| IBIS file stm32mp251_253_255_257_vfbga361.ibs
[IBIS ver] 5.1
[File name] stm32mp251_253_255_257_vfbga361.ibs
[File Rev] 1.3
[Date] 09-10-2025
[Source] Data Created at STMicroelectronics
[Notes]  File originated from ELDO simulations.
[Disclaimer]  This information is for modeling purpose only and is
   not guaranted. The information is subject to change without
   notice.
[Copyright] Copyright 2025 STMicroelectronics Inc.
|   Component stm32mp251_253_255_257_vfbga361
[Component] stm32mp251_253_255_257_vfbga361
[Manufacturer] STMicroelectronics
[Package]
| variable   typ   min   max
R_pkg   0.0   0.0   0.0
L_pkg   0.0H   0.0H   0.0H
C_pkg   0.0F   0.0F   0.0F
[Pin]  signal_name   model_name   R_pin   L_pin   C_pin
A1 VSS gnd
A10 PD2 io8_tt
A11 PD15 io8_tt_i3c
A12 PD6 io8_tt
A13 PD14 io8_tt_i3c
A14 PE2 io8_tt
A15 PE3 io8_tt
A16 PE13 io8_tt
A17 DDR_DQ11 mal4drv27_PAD
A18 DDR_DQ9 mal4drv27_PAD
A19 VSS gnd
A2 DSI_D3P DPHY_IBIS
A3 DSI_D2P DPHY_IBIS
A4 DSI_CKN DPHY_IBIS
A5 DSI_D0N DPHY_IBIS
A6 DSI_D1N DPHY_IBIS
A7 PB8 io8_tt
A8 PB9 io8_tt
A9 PB3 io8_tt
B1 VDDCSI nc
B10 PD11 io8_tt_i3c
B11 B11 nc
B12 PD5 io8_tt
B13 PE0 io8_tt
B14 PE4 io8_tt
B15 PE8 io8_tt
B16 PE11 io8_tt
B17 DDR_DQ10 mal4drv27_PAD
B18 DDR_DQS1N mal4drv27_PAD
B19 DDR_DQS1P mal4drv27_PAD
B2 DSI_D3N DPHY_IBIS
B3 DSI_D2N DPHY_IBIS
B4 DSI_CKP DPHY_IBIS
B5 DSI_D0P DPHY_IBIS
B6 DSI_D1P DPHY_IBIS
B7 PB11 io8_tt
B8 PB0 io8_tt
B9 PB5 io8_tt_i3c
C1 CSI_CKP DPHY_IBIS_L1
C10 PD9 io8_tt
C11 PD0 io8_tt
C12 PD4 io8_tt
C13 PE1 io8_tt
C14 PE5 io8_tt
C15 PE7 io8_tt
C16 PE12 io8_tt
C17 DDR_DQ8 mal4drv27_PAD
C18 DDR_DQ15 mal4drv27_PAD
C19 DDR_DQM1 mal4drv27_PAD
C2 CSI_CKN DPHY_IBIS_L1
C3 VSS gnd
C4 DSI_REXT nc
C5 VDDA18DSI power
C6 VDDDSI nc
C7 VSS gnd
C8 PB6 io8_tt
C9 PB4 io8_tt_i3c
D1 CSI_D1P DPHY_IBIS_L1
D10 VDDIO1 power
D11 PD10 io8_tt_i3c
D12 PD7 io8_tt
D13 VSS gnd
D14 PE15 io8_tt
D15 PE10 io8_tt
D16 VDDA18DDR nc
D17 DDR_DQ14 mal4drv27_PAD
D18 DDR_DQ13 mal4drv27_PAD
D19 DDR_DQ12 mal4drv27_PAD
D2 CSI_D1N DPHY_IBIS_L1
D3 VDDA18CSI power
D4 D4 nc
D5 D5 nc
D6 VDDIO4 power
D7 PB7 io8_tt
D8 PD3 io8_tt
D9 PB1 io8_tt
E1 CSI_D0N DPHY_IBIS_L1
E10 VDDIO3 power
E11 PD8 io8_tt
E12 PB10 io8_tt
E13 VDDCPU nc
E14 PB12 io8_tt
E15 VDDA18PLL1 nc
E16 VSS gnd
E17 DDR_RESETN nc
E18 DDR_A9 mal4drv20_PAD
E19 DDR_A20 mal4drv20_PAD
E2 CSI_D0P DPHY_IBIS_L1
E3 CSI_REXT nc
E4 PG15 io8_tt
E5 PG8 io8_tt
E6 VDDIO4 power
E7 PG7 io8_tt
E8 VSS gnd
E9 PB2 io8_tt
F1 LVDS1_D0N nc
F10 VDDIO3 power
F11 VSS gnd
F12 F12 nc
F13 VSS gnd
F14 PE6 io8_tt
F15 PE9 io8_tt
F16 VDDQDDR power
F17 DDR_A0 mal4drv20_PAD
F18 DDR_A11 mal4drv20_PAD
F19 DDR_A21 mal4drv20_PAD
F2 LVDS1_D0P nc
F3 LVDS1_D1N nc
F4 LVDS1_D1P nc
F5 PG10 io8_tt
F6 VSS gnd
F7 PG11 io8_tt
F8 VDDIO2 power
F9 PD1 io8_tt
G1 G1 nc
G10 VDDCORE nc
G11 VSS gnd
G12 PH4 io8_tt
G13 VDDCPU nc
G14 PE14 io8_tt
G15 PB13 io8_tt
G16 DDR_ZQ nc
G17 DDR_A1 mal4drv20_PAD
G18 DDR_A10 mal4drv20_PAD
G19 DDR_A22 mal4drv20_PAD
G2 PG9 io8_tt
G3 LVDS1_D2N nc
G4 LVDS1_D2P nc
G5 PF15 io8_tt
G6 VDDA18PLL2 nc
G7 PF14 io8_tt
G8 VSS gnd
G9 PD13 io8_tt
H1 PI0 io8_tt
H10 VSS gnd
H11 VDDCORE nc
H12 PG3 io8_tt
H13 VSS gnd
H14 PD12 io8_tt
H15 PB14 io8_tt
H16 VSS gnd
H17 DDR_A25 mal4drv20_PAD
H18 DDR_A8 mal4drv20_PAD
H19 DDR_A23 mal4drv20_PAD
H2 PF13 io8_tt
H3 LVDS1_D4N nc
H4 LVDS1_D4P nc
H5 PG14 io8_tt
H6 VDDA18PLL3 nc
H7 PG12 io8_tt
H8 VDD power
H9 PI3 io8_tt
J1 VDDLVDS nc
J10 VDDCORE nc
J11 VSS gnd
J12 PA5 io8_tt
J13 VDDCPU nc
J14 VSS gnd
J15 PB15 io8_tt
J16 VDDQDDR power
J17 DDR_A2 mal4drv20_PAD
J18 DDR_A13 mal4drv20_PAD
J19 DDR_A3 mal4drv20_PAD
J2 LVDS1_D3N nc
J3 LVDS1_D3P nc
J4 VDDA18LVDS power
J5 PI2 io8_tt
J6 VSS gnd
J7 PG13 io8_tt_i3c
J8 VSS gnd
J9 PI1 io8_tt_i3c
K1 PG5 io8_tt_i3c
K10 VSS gnd
K11 VDDCORE nc
K12 PA9 io8_tt
K13 VSS gnd
K14 PH3 io8_tt_i3c
K15 PA7 io8_tt
K16 VSS gnd
K17 DDR_VREF nc
K18 DDR_A14 mal4drv20_PAD
K19 DDR_A26 mal4drv20_PAD
K2 PG6 io8_tt_i3c
K3 PZ6 io8_tt
K4 VSS gnd
K5 VSS gnd
K6 K6 nc
K7 K7 nc
K8 VDD power
K9 PA8 io8_tt_i3c
L1 PZ7 io8_tt
L10 VDDCORE nc
L11 VSS gnd
L12 PH7 io8_tt_i3c
L13 VDDCPU nc
L14 PH2 io8_tt_i3c
L15 PH6 io8_tt_i3c
L16 VDDQDDR power
L17 DDR_A5 mal4drv20_PAD
L18 DDR_A15 mal4drv20_PAD
L19 DDR_A27 mal4drv20_PAD
L2 PZ9 io8_tt_i3c
L3 PZ8 io8_tt
L4 PZ4 io8_tt_i3c
L5 PZ0 io8_tt_i3c
L6 VDD power
L7 PF12 io8_tt
L8 VSS gnd
L9 PF10 io8_tt
M1 OSC32_OUT isudq_tt
M10 VSS gnd
M11 VDDGPU nc
M12 PH8 io8_tt
M13 VDDCPU nc
M14 PA6 io8_tt
M15 PA10 io8_tt
M16 VDDQDDR power
M17 DDR_A4 mal4drv20_PAD
M18 DDR_A16 mal4drv20_PAD
M19 DDR_A28 mal4drv20_PAD
M2 OSC32_IN isudq_tt
M3 PZ2 io8_tt_i3c
M4 PZ1 io8_tt_i3c
M5 PZ3 io8_tt_i3c
M6 M6 nc
M7 PG2 io8_tt_i3c
M8 V08CAP nc
M9 PH5 io8_tt
N1 PDR_ON nc
N10 VDDCORE nc
N11 VSS gnd
N12 PA2 io8_tt_i3c
N13 VSS gnd
N14 VDDGPU nc
N15 PA1 io8_tt_i3c
N16 VSS gnd
N17 DDR_A6 mal4drv20_PAD
N18 DDR_A17 mal4drv20_PAD
N19 DDR_A29 mal4drv20_PAD
N2 LVDS2_D1P nc
N3 PZ5 io8_tt
N4 N4 nc
N5 VDDA18AON power
N6 VDDA18ADC nc
N7 PG4 io8_tt
N8 VDDCORE nc
N9 PF0 io8_tt_i3c
P1 PWR_LP io8_tt
P10 VSS gnd
P11 VDDGPU nc
P12 PA4 io8_tt
P13 VDDGPU nc
P14 VSS gnd
P15 PA0 io8_tt
P16 VDDQDDR power
P17 DDR_A7 mal4drv20_PAD
P18 DDR_A18 mal4drv20_PAD
P19 DDR_A30 mal4drv20_PAD
P2 PWR_CPU_ON io8_tt
P3 BOOT1 isudq_tt
P4 PC13 io8_tt
P5 ANA1 nc
P6 VSSA gnd
P7 PF5 io8_tt
P8 VSS gnd
P9 PF2 io8_tt_i3c
R1 OSC_IN isudq_tt
R10 VDDGPU nc
R11 VSS gnd
R12 PA3 io8_tt_i3c
R13 VDDA18COMBOPHY power
R14 VDD33USB power
R15 USB3DR_TXRTUNE nc
R16 VSS gnd
R17 DDR_A12 mal4drv20_PAD
R18 VSS gnd
R19 DDR_A31 mal4drv20_PAD
R2 OSC_OUT isudq_tt
R3 BOOT3 isudq_tt
R4 PG1 io8_tt_i3c
R5 ANA0 nc
R6 VBAT power
R7 PC6 io8_tt_i3c
R8 PA12 io8_tt_i3c
R9 PA11 io8_tt
T1 LVDS2_D2N io8_tt
T10 PA15 io8_tt_i3c
T11 PH11 io8_tt
T12 USB3DR_VBUS nc
T13 VDDA18USB power
T14 VDDCOMBOPHY nc
T15 USBH_HS_TXRTUNE nc
T16 VDDQDDR power
T17 DDR_DQM0 mal4drv27_PAD
T18 DDR_DQ5 mal4drv27_PAD
T19 DDR_DQ4 mal4drv27_PAD
T2 BOOT0 isudq_tt
T3 BOOT2 isudq_tt
T4 PF11 io8_tt
T5 PG0 io8_tt_i3c
T6 PF9 io8_tt
T7 PC5 io8_tt_i3c
T8 PA14 io8_tt
T9 PC2 io8_tt
U1 VREFN nc
U10 PH10 io8_tt
U11 VDD33UCPD nc
U12 VDDPCIECLK nc
U13 PCIE_CLKINP nc
U14 PCIE_CLKOUTP nc
U15 COMBOPHY_TX1P synopsys_usb3_tx
U16 COMBOPHY_RX1P synopsys_usb3_rx
U17 DDR_DQ3 mal4drv27_PAD
U18 DDR_DQ7 mal4drv27_PAD
U19 DDR_DQ6 mal4drv27_PAD
U2 VREFP nc
U3 PWR_ON io8_tt
U4 PC3 io8_tt
U5 PF6 io8_tt
U6 PC8 io8_tt
U7 PF8 io8_tt
U8 PF1 io8_tt
U9 PH13 io8_tt
V1 JTDO-TRACESWO io8_tt
V10 PC1 io8_tt_i3c
V11 USBH_HS_DM USB2_HS_IBIS
V12 USB3DR_DM USB2_HS_IBIS
V13 PCIE_CLKINN nc
V14 PCIE_CLKOUTN nc
V15 COMBOPHY_TX1N synopsys_usb3_tx
V16 COMBOPHY_RX1N synopsys_usb3_rx
V17 DDR_DQ2 mal4drv27_PAD
V18 DDR_DQS0N mal4drv27_PAD
V19 DDR_DQS0P mal4drv27_PAD
V2 LVDS2_D1N io8_tt
V3 PC4 io8_tt
V4 PC12 io8_tt_i3c
V5 PC11 io8_tt
V6 PC9 io8_tt
V7 PF7 io8_tt
V8 PH12 io8_tt
V9 PC0 io8_tt
W1 VSS gnd
W10 PF3 io8_tt
W11 USBH_HS_DP USB2_HS_IBIS
W12 USB3DR_DP USB2_HS_IBIS
W13 UCPD1_CC1 nc
W14 UCPD1_CC2 nc
W15 COMBOPHY_REXT nc
W16 VDDCOMBOPHYTX nc
W17 DDR_DQ1 mal4drv27_PAD
W18 DDR_DQ0 mal4drv27_PAD
W19 VSS gnd
W2 JTMS-SWDIO io8_tt
W3 JTDI io8_tt
W4 JTCK-SWCLK io8_tt
W5 PC7 io8_tt
W6 PC10 io8_tt
W7 PF4 io8_tt
W8 PH9 io8_tt
W9 PA13 io8_tt
[Package Model]   10x10_bot
[Pin Mapping]   pulldown_ref   pullup_ref   | Comment
A1 gnd nc
A10 gnd VDDIO3
A11 gnd VDD
A12 gnd VDDIO3
A13 gnd VDD
A14 gnd VDDIO1
A15 gnd VDDIO1
A16 gnd VDDIO2
A17 gnd VDDQDDR
A18 gnd VDDQDDR
A19 gnd nc
A2 gnd VDDA18DSI
A3 gnd VDDA18DSI
A4 gnd VDDA18DSI
A5 gnd VDDA18DSI
A6 gnd VDDA18DSI
A7 gnd VDDIO4
A8 gnd VDDIO4
A9 gnd VDDIO4
B1 nc nc
B10 gnd VDDIO3
B11 nc nc
B12 gnd VDDIO3
B13 gnd VDDIO1
B14 gnd VDDIO1
B15 gnd VDDIO2
B16 gnd VDDIO2
B17 gnd VDDQDDR
B18 gnd VDDQDDR
B19 gnd VDDQDDR
B2 gnd VDDA18DSI
B3 gnd VDDA18DSI
B4 gnd VDDA18DSI
B5 gnd VDDA18DSI
B6 gnd VDDA18DSI
B7 gnd VDDIO4
B8 gnd VDDIO4
B9 gnd VDDIO4
C1 gnd  VDDA18CSI
C10 gnd VDDIO3
C11 gnd VDDIO3
C12 gnd VDDIO3
C13 gnd VDDIO1
C14 gnd VDDIO1
C15 gnd VDDIO2
C16 gnd VDDIO2
C17 gnd VDDQDDR
C18 gnd VDDQDDR
C19 gnd VDDQDDR
C2 gnd  VDDA18CSI
C3 gnd nc
C4 nc nc
C5 nc VDDA18DSI
C6 nc nc
C7 gnd nc
C8 gnd VDDIO4
C9 gnd VDDIO4
D1 gnd  VDDA18CSI
D10 nc VDDIO1
D11 gnd VDDIO3
D12 gnd VDDIO3
D13 gnd nc
D14 gnd VDDIO2
D15 gnd VDDIO2
D16 nc nc
D17 gnd VDDQDDR
D18 gnd VDDQDDR
D19 gnd VDDQDDR
D2 gnd  VDDA18CSI
D3 nc VDDA18CSI
D4 nc nc
D5 nc nc
D6 nc VDDIO4
D7 gnd VDDIO4
D8 gnd VDDIO3
D9 gnd VDDIO4
E1 gnd  VDDA18CSI
E10 nc VDDIO3
E11 gnd VDDIO3
E12 gnd VDDIO4
E13 nc nc
E14 gnd VDD
E15 nc nc
E16 gnd nc
E17 nc nc
E18 gnd VDDQDDR
E19 gnd VDDQDDR
E2 gnd  VDDA18CSI
E3 nc nc
E4 gnd VDD
E5 gnd VDD
E6 nc VDDIO4
E7 gnd VDD
E8 gnd nc
E9 gnd VDDIO4
F1 nc nc
F10 nc VDDIO3
F11 gnd nc
F12 nc nc
F13 gnd nc
F14 gnd VDDIO2
F15 gnd VDDIO2
F16 nc VDDQDDR
F17 gnd VDDQDDR
F18 gnd VDDQDDR
F19 gnd VDDQDDR
F2 nc nc
F3 nc nc
F4 nc nc
F5 gnd VDD
F6 gnd nc
F7 gnd VDD
F8 nc VDDIO2
F9 gnd VDDIO3
G1 nc nc
G10 nc nc
G11 gnd nc
G12 gnd VDD
G13 nc nc
G14 gnd VDDIO2
G15 gnd VDD
G16 nc nc
G17 gnd VDDQDDR
G18 gnd VDDQDDR
G19 gnd VDDQDDR
G2 gnd VDD
G3 nc nc
G4 nc nc
G5 gnd VDD
G6 nc nc
G7 gnd VDD
G8 gnd nc
G9 gnd VDD
H1 gnd VDD
H10 gnd nc
H11 nc nc
H12 gnd VDD  | Depending on IO usage
| H12 gnd  VSW  | Depending on IO usage
H13 gnd nc
H14 gnd VDD
H15 gnd VDD
H16 gnd nc
H17 gnd VDDQDDR
H18 gnd VDDQDDR
H19 gnd VDDQDDR
H2 gnd VDD
H3 nc nc
H4 nc nc
H5 gnd VDD
H6 nc nc
H7 gnd VDD
H8 nc VDD
H9 gnd VDD
J1 nc nc
J10 nc nc
J11 gnd nc
J12 gnd VDD
J13 nc nc
J14 gnd nc
J15 gnd VDD
J16 nc VDDQDDR
J17 gnd VDDQDDR
J18 gnd VDDQDDR
J19 gnd VDDQDDR
J2 nc nc
J3 nc nc
J4 nc VDDA18LVDS
J5 gnd VDD
J6 gnd nc
J7 gnd VDD
J8 gnd nc
J9 gnd VDD
K1 gnd VDD
K10 gnd nc
K11 nc nc
K12 gnd VDD
K13 gnd nc
K14 gnd VDD
K15 gnd VDD
K16 gnd nc
K17 nc nc
K18 gnd VDDQDDR
K19 gnd VDDQDDR
K2 gnd VDD
K3 gnd VDD  | Depending on IO usage
| K3 gnd  VSW  | Depending on IO usage
K4 gnd nc
K5 gnd nc
K6 nc nc
K7 nc nc
K8 nc VDD
K9 gnd VDD
L1 gnd VDD
L10 nc nc
L11 gnd nc
L12 gnd VDD
L13 nc nc
L14 gnd VDD
L15 gnd VDD
L16 nc VDDQDDR
L17 gnd VDDQDDR
L18 gnd VDDQDDR
L19 gnd VDDQDDR
L2 gnd VDD
L3 gnd VDD
L4 gnd VDD  | Depending on IO usage
| L4 gnd  VSW  | Depending on IO usage
L5 gnd VDD  | Depending on IO usage
| L5 gnd  VSW  | Depending on IO usage
L6 nc VDD
L7 gnd VDD
L8 gnd nc
L9 gnd VDD
M1 gnd VSW
M10 gnd nc
M11 nc nc
M12 gnd VDD
M13 nc nc
M14 gnd VDD
M15 gnd VDD
M16 nc VDDQDDR
M17 gnd VDDQDDR
M18 gnd VDDQDDR
M19 gnd VDDQDDR
M2 gnd VSW
M3 gnd VDD  | Depending on IO usage
| M3 gnd  VSW  | Depending on IO usage
M4 gnd VDD  | Depending on IO usage
| M4 gnd  VSW  | Depending on IO usage
M5 gnd VDD  | Depending on IO usage
| M5 gnd  VSW  | Depending on IO usage
M6 nc nc
M7 gnd VDD
M8 nc nc
M9 gnd VDD
N1 nc nc
N10 nc nc
N11 gnd nc
N12 gnd VDD
N13 gnd nc
N14 nc nc
N15 gnd VDD
N16 gnd nc
N17 gnd VDDQDDR
N18 gnd VDDQDDR
N19 gnd VDDQDDR
N2 nc nc
N3 gnd VDD  | Depending on IO usage
| N3 gnd  VSW  | Depending on IO usage
N4 nc nc
N5 nc VDDA18AON
N6 nc nc
N7 gnd VDD
N8 nc nc
N9 gnd VDD
P1 gnd VDD
P10 gnd nc
P11 nc nc
P12 gnd VDD
P13 nc nc
P14 gnd nc
P15 gnd VDD
P16 nc VDDQDDR
P17 gnd VDDQDDR
P18 gnd VDDQDDR
P19 gnd VDDQDDR
P2 gnd VDD
P3 gnd VDD
P4 gnd VSW
P5 nc nc
P6 gnd nc
P7 gnd VDD
P8 gnd nc
P9 gnd VDD
R1 gnd VDDA18AON
R10 nc nc
R11 gnd nc
R12 gnd VDD
R13 nc VDDA18COMBOPHY
R14 nc VDD33USB
R15 nc nc
R16 gnd nc
R17 gnd VDDQDDR
R18 gnd nc
R19 gnd VDDQDDR
R2 gnd VDDA18AON
R3 gnd VDD
R4 gnd VDD  | Depending on IO usage
| R4 gnd  VSW  | Depending on IO usage
R5 nc nc
R6 nc VSW
R7 gnd VDD
R8 gnd VDD
R9 gnd VDD
T1 gnd VDD
T10 gnd VDD
T11 gnd VDD
T12 nc nc
T13 nc VDDA18USB
T14 nc nc
T15 nc nc
T16 nc VDDQDDR
T17 gnd VDDQDDR
T18 gnd VDDQDDR
T19 gnd VDDQDDR
T2 gnd VDD
T3 gnd VDD
T4 gnd VDD
T5 gnd VDD
T6 gnd VDD
T7 gnd VDD  | Depending on IO usage
| T7 gnd  VSW  | Depending on IO usage
T8 gnd VDD
T9 gnd VDD
U1 nc nc
U10 gnd VDD
U11 nc nc
U12 nc nc
U13 nc nc
U14 nc nc
U15 gnd VDDA18COMBOPHY
U16 gnd VDDA18COMBOPHY
U17 gnd VDDQDDR
U18 gnd VDDQDDR
U19 gnd VDDQDDR
U2 nc nc
U3 gnd VDD
U4 gnd VDD  | Depending on IO usage
| U4 gnd  VSW  | Depending on IO usage
U5 gnd VDD  | Depending on IO usage
| U5 gnd  VSW  | Depending on IO usage
U6 gnd VDD
U7 gnd VDD
U8 gnd VDD
U9 gnd VDD
V1 gnd VDD
V10 gnd VDD
V11 gnd VDD33USB
V12 gnd VDD33USB
V13 nc nc
V14 nc nc
V15 gnd VDDA18COMBOPHY
V16 gnd VDDA18COMBOPHY
V17 gnd VDDQDDR
V18 gnd VDDQDDR
V19 gnd VDDQDDR
V2 gnd VDD
V3 gnd VDD  | Depending on IO usage
| V3 gnd  VSW  | Depending on IO usage
V4 gnd VDD
V5 gnd VDD
V6 gnd VDD
V7 gnd VDD  | Depending on IO usage
| V7 gnd  VSW  | Depending on IO usage
V8 gnd VDD
V9 gnd VDD
W1 gnd nc
W10 gnd VDD
W11 gnd VDD33USB
W12 gnd VDD33USB
W13 nc nc
W14 nc nc
W15 nc nc
W16 nc nc
W17 gnd VDDQDDR
W18 gnd VDDQDDR
W19 gnd nc
W2 gnd VDD
W3 gnd VDD
W4 gnd VDD
W5 gnd VDD
W6 gnd VDD
W7 gnd VDD
W8 gnd VDD
W9 gnd VDD
[Diff Pin]  inv_pin  vdiff  tdelay_typ  tdelay_min  tdelay_max
M17  L17  0.320V 0ns  NA  NA  |CK
V19  V18  0.320V 0ns  NA  NA  |DQS0
B19  B18  0.320V 0ns  NA  NA  |DQS1
B4   A4   NA   NA   NA   NA  |DSI CKP CKN
B5   A5   400.000mV   0ns   NA   NA   |D0P D0N
B6   A6   400.000mV   0ns   NA   NA   |D1P D1N
B3   A3   400.000mV   0ns   NA   NA   |D2P D2N
A2   B2   400.000mV   0ns   NA   NA   |D3P D3N
W12   V12   NA   NA   NA   NA   |USB3DR_DP _DM
W11   V11   NA   NA   NA   NA   |USBH_HS_DP _DM
[Model Selector] DPHY_IBIS_L1
DPHY_RX_2P5G_L1   DPHY HSRX model at 2.5Gbps for lane 1
DPHY_RX_1P5G_L1   DPHY HSRX model at 1.5Gbps for lane 1
[Model Selector] DPHY_IBIS
DPHY_TX_2P5G   DPHY HSTX model at 2.5Gbps
DPHY_TX_1P5G   DPHY HSTX model at 1.5Gbps
[Model Selector] USB2_HS_IBIS
USB2_HSRX   USB2 HSRX model
USB2_HSTX_00_0_01_0011_11   TuningBits_AMP_PULSE_RISE_REF_XV=00_0_01_0011_11
USB2_HSTX_00_0_10_0101_11   TuningBits_AMP_PULSE_RISE_REF_XV=00_0_10_0101_11
USB2_HSTX_00_0_11_0111_11   TuningBits_AMP_PULSE_RISE_REF_XV=00_0_11_0111_11
USB2_HSTX_00_1_01_0011_11   TuningBits_AMP_PULSE_RISE_REF_XV=00_1_01_0011_11
USB2_HSTX_00_1_10_0101_11   TuningBits_AMP_PULSE_RISE_REF_XV=00_1_10_0101_11
USB2_HSTX_00_1_11_0111_11   TuningBits_AMP_PULSE_RISE_REF_XV=00_1_11_0111_11
USB2_HSTX_01_0_01_0011_11   TuningBits_AMP_PULSE_RISE_REF_XV=01_0_01_0011_11
USB2_HSTX_01_0_10_0101_11   TuningBits_AMP_PULSE_RISE_REF_XV=01_0_10_0101_11
USB2_HSTX_01_0_11_0111_11   TuningBits_AMP_PULSE_RISE_REF_XV=01_0_11_0111_11
USB2_HSTX_01_1_01_0011_11   TuningBits_AMP_PULSE_RISE_REF_XV=01_1_01_0011_11
USB2_HSTX_01_1_10_0101_11   TuningBits_AMP_PULSE_RISE_REF_XV=01_1_10_0101_11
USB2_HSTX_01_1_11_0111_11   TuningBits_AMP_PULSE_RISE_REF_XV=01_1_11_0111_11
USB2_HSTX_10_0_01_0011_11   TuningBits_AMP_PULSE_RISE_REF_XV=10_0_01_0011_11
USB2_HSTX_10_0_10_0101_11   TuningBits_AMP_PULSE_RISE_REF_XV=10_0_10_0101_11
USB2_HSTX_10_0_11_0111_11   TuningBits_AMP_PULSE_RISE_REF_XV=10_0_11_0111_11
USB2_HSTX_10_1_01_0011_11   TuningBits_AMP_PULSE_RISE_REF_XV=10_1_01_0011_11
USB2_HSTX_10_1_10_0101_11   TuningBits_AMP_PULSE_RISE_REF_XV=10_1_10_0101_11
USB2_HSTX_10_1_11_0111_11   TuningBits_AMP_PULSE_RISE_REF_XV=10_1_11_0111_11
[Model Selector] io8_tt
io8_tt_ls_3v3   "GPIO - 3V tolerant - 3.3V range - Low speed"
io8_tt_ms_3v3   "GPIO - 3V tolerant - 3.3V range - Med speed"
io8_tt_fs_3v3   "GPIO - 3V tolerant - 3.3V range - Fast speed"
io8_tt_hs_3v3   "GPIO - 3V tolerant - 3.3V range - High speed"
io8_tt_hslv_ls_1v8   "GPIO HSLV - 3V tolerant - 1.8V range - Low speed"
io8_tt_hslv_ms_1v8   "GPIO HSLV - 3V tolerant - 1.8V range - Med speed"
io8_tt_hslv_fs_1v8   "GPIO HSLV - 3V tolerant - 1.8V range - Fast speed"
io8_tt_hslv_hs_1v8   "GPIO HSLV - 3V tolerant - 1.8V range - High speed"
[Model Selector] io8_tt_i3c
io8_tt_ls_3v3   "GPIO - 3V tolerant - 3.3V range - Low speed"
io8_tt_ms_3v3   "GPIO - 3V tolerant - 3.3V range - Med speed"
io8_tt_fs_3v3   "GPIO - 3V tolerant - 3.3V range - Fast speed"
io8_tt_hs_3v3   "GPIO - 3V tolerant - 3.3V range - High speed"
io8_tt_hslv_ls_1v8   "GPIO HSLV - 3V tolerant - 1.8V range - Low speed"
io8_tt_hslv_ms_1v8   "GPIO HSLV - 3V tolerant - 1.8V range - Med speed"
io8_tt_hslv_fs_1v8   "GPIO HSLV - 3V tolerant - 1.8V range - Fast speed"
io8_tt_hslv_hs_1v8   "GPIO HSLV - 3V tolerant - 1.8V range - High speed"
io8_tt_i3c_3v3   "GPIO - 3V tolerant - 3.3V range - Open drain"
[Model Selector] isudq_tt
isudq_tt_1v8   "Input Buffer - 3V tolerant - 1.8V range"
isudq_tt_3v3   "Input Buffer - 3V tolerant - 3.3V range"
[Model Selector]   mal4drv20_PAD
mal4drv20_d3l_40   DDR3L mal4drv20 cell  Z0=40-Ohm Driver
mal4drv20_d3l_60   DDR3L mal4drv20 cell  Z0=60-Ohm Driver
mal4drv20_d3l_120   DDR3L mal4drv20 cell  Z0=120-Ohm Driver
mal4drv20_d3_20   DDR3 mal4drv20 cell  Z0=20-Ohm Driver
mal4drv20_d3_24   DDR3 mal4drv20 cell  Z0=24-Ohm Driver
mal4drv20_d3_30   DDR3 mal4drv20 cell  Z0=30-Ohm Driver
mal4drv20_d3_40   DDR3 mal4drv20 cell  Z0=40-Ohm Driver
mal4drv20_d3_60   DDR3 mal4drv20 cell  Z0=60-Ohm Driver
mal4drv20_d4_20   DDR4 mal4drv20 cell  Z0=20-Ohm Driver
mal4drv20_d4_24   DDR4 mal4drv20 cell  Z0=24-Ohm Driver
mal4drv20_d4_30   DDR4 mal4drv20 cell  Z0=30-Ohm Driver
mal4drv20_d4_40   DDR4 mal4drv20 cell  Z0=40-Ohm Driver
mal4drv20_d4_60   DDR4 mal4drv20 cell  Z0=60-Ohm Driver
mal4drv20_dl4_20   LPDDR4 mal4drv20 cell  Z0=20-Ohm Driver
mal4drv20_dl4_24   LPDDR4 mal4drv20 cell  Z0=24-Ohm Driver
mal4drv20_dl4_30   LPDDR4 mal4drv20 cell  Z0=30-Ohm Driver
mal4drv20_dl4_40   LPDDR4 mal4drv20 cell  Z0=40-Ohm Driver
mal4drv20_dl4_60   LPDDR4 mal4drv20 cell  Z0=60-Ohm Driver
[Model Selector]   mal4drv27_PAD
mal4drv27_d3l_40   DDR3L mal4drv27 cell  Z0=40-Ohm Driver
mal4drv27_d3l_48   DDR3L mal4drv27 cell  Z0=48-Ohm Driver
mal4drv27_d3l_60   DDR3L mal4drv27 cell  Z0=60-Ohm Driver
mal4drv27_d3l_80   DDR3L mal4drv27 cell  Z0=80-Ohm Driver
mal4drv27_d3l_120   DDR3L mal4drv27 cell  Z0=120-Ohm Driver
mal4drv27_d3l_240   DDR3L mal4drv27 cell  Z0=240-Ohm Driver
mal4drv27_d3l_odt120   DDR3L mal4drv27 cell 120-Ohm ODT Receiver
mal4drv27_d3l_odt60   DDR3L mal4drv27 cell 60-Ohm ODT Receiver
mal4drv27_d3l_odtoff   DDR3L mal4drv27 cell ODT OFF Receiver
mal4drv27_d3_28   DDR3 mal4drv27 cell  Z0=28-Ohm Driver
mal4drv27_d3_34   DDR3 mal4drv27 cell  Z0=34-Ohm Driver
mal4drv27_d3_40   DDR3 mal4drv27 cell  Z0=40-Ohm Driver
mal4drv27_d3_53   DDR3 mal4drv27 cell  Z0=53-Ohm Driver
mal4drv27_d3_odt120   DDR3 mal4drv27 cell 120-Ohm ODT Receiver
mal4drv27_d3_odt60   DDR3 mal4drv27 cell 60-Ohm ODT Receiver
mal4drv27_d4_28   DDR4 mal4drv27 cell  Z0=28-Ohm Driver
mal4drv27_d4_34   DDR4 mal4drv27 cell  Z0=34-Ohm Driver
mal4drv27_d4_40   DDR4 mal4drv27 cell  Z0=40-Ohm Driver
mal4drv27_d4_53   DDR4 mal4drv27 cell  Z0=53-Ohm Driver
mal4drv27_d4_odt120   DDR4 mal4drv27 cell 120-Ohm ODT Receiver
mal4drv27_d4_odt240   DDR4 mal4drv27 cell 240-Ohm ODT Receiver
mal4drv27_d4_odt48   DDR4 mal4drv27 cell 48-Ohm ODT Receiver
mal4drv27_d4_odt60   DDR4 mal4drv27 cell 60-Ohm ODT Receiver
mal4drv27_d4_odt80   DDR4 mal4drv27 cell 80-Ohm ODT Receiver
mal4drv27_dl4_28   LPDDR4 mal4drv27 cell  Z0=28-Ohm Driver
mal4drv27_dl4_34   LPDDR4 mal4drv27 cell  Z0=34-Ohm Driver
mal4drv27_dl4_40   LPDDR4 mal4drv27 cell  Z0=40-Ohm Driver
mal4drv27_dl4_53   LPDDR4 mal4drv27 cell  Z0=53-Ohm Driver
mal4drv27_dl4_odt48   LPDDR4 mal4drv27 cell 48-Ohm ODT Receiver
mal4drv27_dl4_odt60   LPDDR4 mal4drv27 cell 60-Ohm ODT Receiver
[Define Package Model]  10x10_bot
[Manufacturer]   unknown
[OEM]   unknown
[Description]   unknown
[Number Of Pins]   299
[Pin Numbers]
| Pin Name Terminal   Net Name   Starting Node   Ending Node
   T2   |   1   BOOT0  PANTHER_TOP_CTE_DIE_BUMP_0_97  BGA10X10_BGA_T2
   P3   |   2   BOOT1  PANTHER_TOP_CTE_DIE_BUMP_0_72  BGA10X10_BGA_P3
   T3   |   3   BOOT2  PANTHER_TOP_CTE_DIE_BUMP_0_22  BGA10X10_BGA_T3
   R3   |   4   BOOT3  PANTHER_TOP_CTE_DIE_BUMP_0_122  BGA10X10_BGA_R3
   W15   |   5   COMBOPHY_REXT  PANTHER_TOP_CTE_DIE_BUMP_0_52  BGA10X10_BGA_W15
   V16   |   6   COMBOPHY_RX1N  PANTHER_TOP_CTE_DIE_BUMP_0_125  BGA10X10_BGA_V16
   U16   |   7   COMBOPHY_RX1P  PANTHER_TOP_CTE_DIE_BUMP_0_100  BGA10X10_BGA_U16
   V15   |   8   COMBOPHY_TX1N  PANTHER_TOP_CTE_DIE_BUMP_0_51  BGA10X10_BGA_V15
   U15   |   9   COMBOPHY_TX1P  PANTHER_TOP_CTE_DIE_BUMP_0_75  BGA10X10_BGA_U15
   C2   |   10   CSI_CKN  PANTHER_TOP_CTE_DIE_BUMP_0_406  BGA10X10_BGA_C2
   C1   |   11   CSI_CKP  PANTHER_TOP_CTE_DIE_BUMP_0_448  BGA10X10_BGA_C1
   E1   |   12   CSI_D0N  PANTHER_TOP_CTE_DIE_BUMP_0_426  BGA10X10_BGA_E1
   E2   |   13   CSI_D0P  PANTHER_TOP_CTE_DIE_BUMP_0_384  BGA10X10_BGA_E2
   D2   |   14   CSI_D1N  PANTHER_TOP_CTE_DIE_BUMP_0_385  BGA10X10_BGA_D2
   D1   |   15   CSI_D1P  PANTHER_TOP_CTE_DIE_BUMP_0_427  BGA10X10_BGA_D1
   E3   |   16   CSI_REXT  PANTHER_TOP_CTE_DIE_BUMP_0_489  BGA10X10_BGA_E3
   F17   |   17   DDR_A0  PANTHER_TOP_CTE_DIE_BUMP_0_240  BGA10X10_BGA_F17
   G17   |   18   DDR_A1  PANTHER_TOP_CTE_DIE_BUMP_0_244  BGA10X10_BGA_G17
   J17   |   19   DDR_A2  PANTHER_TOP_CTE_DIE_BUMP_0_242  BGA10X10_BGA_J17
   J19   |   20   DDR_A3  PANTHER_TOP_CTE_DIE_BUMP_0_245  BGA10X10_BGA_J19
   M17   |   21   DDR_A4  PANTHER_TOP_CTE_DIE_BUMP_0_250  BGA10X10_BGA_M17
   L17   |   22   DDR_A5  PANTHER_TOP_CTE_DIE_BUMP_0_248  BGA10X10_BGA_L17
   N17   |   23   DDR_A6  PANTHER_TOP_CTE_DIE_BUMP_0_253  BGA10X10_BGA_N17
   P17   |   24   DDR_A7  PANTHER_TOP_CTE_DIE_BUMP_0_252  BGA10X10_BGA_P17
   H18   |   25   DDR_A8  PANTHER_TOP_CTE_DIE_BUMP_0_256  BGA10X10_BGA_H18
   E18   |   26   DDR_A9  PANTHER_TOP_CTE_DIE_BUMP_0_258  BGA10X10_BGA_E18
   G18   |   27   DDR_A10  PANTHER_TOP_CTE_DIE_BUMP_0_261  BGA10X10_BGA_G18
   F18   |   28   DDR_A11  PANTHER_TOP_CTE_DIE_BUMP_0_260  BGA10X10_BGA_F18
   R17   |   29   DDR_A12  PANTHER_TOP_CTE_DIE_BUMP_0_264  BGA10X10_BGA_R17
   J18   |   30   DDR_A13  PANTHER_TOP_CTE_DIE_BUMP_0_266  BGA10X10_BGA_J18
   K18   |   31   DDR_A14  PANTHER_TOP_CTE_DIE_BUMP_0_268  BGA10X10_BGA_K18
   L18   |   32   DDR_A15  PANTHER_TOP_CTE_DIE_BUMP_0_272  BGA10X10_BGA_L18
   M18   |   33   DDR_A16  PANTHER_TOP_CTE_DIE_BUMP_0_285  BGA10X10_BGA_M18
   N18   |   34   DDR_A17  PANTHER_TOP_CTE_DIE_BUMP_0_284  BGA10X10_BGA_N18
   P18   |   35   DDR_A18  PANTHER_TOP_CTE_DIE_BUMP_0_288  BGA10X10_BGA_P18
   E19   |   36   DDR_A20  PANTHER_TOP_CTE_DIE_BUMP_0_293  BGA10X10_BGA_E19
   F19   |   37   DDR_A21  PANTHER_TOP_CTE_DIE_BUMP_0_292  BGA10X10_BGA_F19
   G19   |   38   DDR_A22  PANTHER_TOP_CTE_DIE_BUMP_0_296  BGA10X10_BGA_G19
   H19   |   39   DDR_A23  PANTHER_TOP_CTE_DIE_BUMP_0_298  BGA10X10_BGA_H19
   H17   |   40   DDR_A25  PANTHER_TOP_CTE_DIE_BUMP_0_301  BGA10X10_BGA_H17
   K19   |   41   DDR_A26  PANTHER_TOP_CTE_DIE_BUMP_0_304  BGA10X10_BGA_K19
   L19   |   42   DDR_A27  PANTHER_TOP_CTE_DIE_BUMP_0_308  BGA10X10_BGA_L19
   M19   |   43   DDR_A28  PANTHER_TOP_CTE_DIE_BUMP_0_306  BGA10X10_BGA_M19
   N19   |   44   DDR_A29  PANTHER_TOP_CTE_DIE_BUMP_0_309  BGA10X10_BGA_N19
   P19   |   45   DDR_A30  PANTHER_TOP_CTE_DIE_BUMP_0_312  BGA10X10_BGA_P19
   R19   |   46   DDR_A31  PANTHER_TOP_CTE_DIE_BUMP_0_314  BGA10X10_BGA_R19
   W18   |   47   DDR_DQ0  PANTHER_TOP_CTE_DIE_BUMP_0_200  BGA10X10_BGA_W18
   W17   |   48   DDR_DQ1  PANTHER_TOP_CTE_DIE_BUMP_0_202  BGA10X10_BGA_W17
   V17   |   49   DDR_DQ2  PANTHER_TOP_CTE_DIE_BUMP_0_175  BGA10X10_BGA_V17
   U17   |   50   DDR_DQ3  PANTHER_TOP_CTE_DIE_BUMP_0_176  BGA10X10_BGA_U17
   T19   |   51   DDR_DQ4  PANTHER_TOP_CTE_DIE_BUMP_0_212  BGA10X10_BGA_T19
   T18   |   52   DDR_DQ5  PANTHER_TOP_CTE_DIE_BUMP_0_216  BGA10X10_BGA_T18
   U19   |   53   DDR_DQ6  PANTHER_TOP_CTE_DIE_BUMP_0_213  BGA10X10_BGA_U19
   U18   |   54   DDR_DQ7  PANTHER_TOP_CTE_DIE_BUMP_0_208  BGA10X10_BGA_U18
   C17   |   55   DDR_DQ8  PANTHER_TOP_CTE_DIE_BUMP_0_234  BGA10X10_BGA_C17
   A18   |   56   DDR_DQ9  PANTHER_TOP_CTE_DIE_BUMP_0_232  BGA10X10_BGA_A18
   B17   |   57   DDR_DQ10  PANTHER_TOP_CTE_DIE_BUMP_0_237  BGA10X10_BGA_B17
   A17   |   58   DDR_DQ11  PANTHER_TOP_CTE_DIE_BUMP_0_236  BGA10X10_BGA_A17
   D19   |   59   DDR_DQ12  PANTHER_TOP_CTE_DIE_BUMP_0_218  BGA10X10_BGA_D19
   D18   |   60   DDR_DQ13  PANTHER_TOP_CTE_DIE_BUMP_0_224  BGA10X10_BGA_D18
   D17   |   61   DDR_DQ14  PANTHER_TOP_CTE_DIE_BUMP_0_220  BGA10X10_BGA_D17
   C18   |   62   DDR_DQ15  PANTHER_TOP_CTE_DIE_BUMP_0_221  BGA10X10_BGA_C18
   T17   |   63   DDR_DQM0  PANTHER_TOP_CTE_DIE_BUMP_0_210  BGA10X10_BGA_T17
   C19   |   64   DDR_DQM1  PANTHER_TOP_CTE_DIE_BUMP_0_229  BGA10X10_BGA_C19
   V18   |   65   DDR_DQS0N  PANTHER_TOP_CTE_DIE_BUMP_0_204  BGA10X10_BGA_V18
   V19   |   66   DDR_DQS0P  PANTHER_TOP_CTE_DIE_BUMP_0_205  BGA10X10_BGA_V19
   B18   |   67   DDR_DQS1N  PANTHER_TOP_CTE_DIE_BUMP_0_228  BGA10X10_BGA_B18
   B19   |   68   DDR_DQS1P  PANTHER_TOP_CTE_DIE_BUMP_0_226  BGA10X10_BGA_B19
   E17   |   69   DDR_RESETN  PANTHER_TOP_CTE_DIE_BUMP_0_269  BGA10X10_BGA_E17
   K17   |   70   DDR_VREF  PANTHER_TOP_CTE_DIE_BUMP_0_280  BGA10X10_BGA_K17
   G16   |   71   DDR_ZQ  PANTHER_TOP_CTE_DIE_BUMP_0_276  BGA10X10_BGA_G16
   A4   |   72   DSI_CKN  PANTHER_TOP_CTE_DIE_BUMP_0_382  BGA10X10_BGA_A4
   B4   |   73   DSI_CKP  PANTHER_TOP_CTE_DIE_BUMP_0_424  BGA10X10_BGA_B4
   A5   |   74   DSI_D0N  PANTHER_TOP_CTE_DIE_BUMP_0_423  BGA10X10_BGA_A5
   B5   |   75   DSI_D0P  PANTHER_TOP_CTE_DIE_BUMP_0_381  BGA10X10_BGA_B5
   A6   |   76   DSI_D1N  PANTHER_TOP_CTE_DIE_BUMP_0_445  BGA10X10_BGA_A6
   B6   |   77   DSI_D1P  PANTHER_TOP_CTE_DIE_BUMP_0_403  BGA10X10_BGA_B6
   B3   |   78   DSI_D2N  PANTHER_TOP_CTE_DIE_BUMP_0_446  BGA10X10_BGA_B3
   A3   |   79   DSI_D2P  PANTHER_TOP_CTE_DIE_BUMP_0_404  BGA10X10_BGA_A3
   B2   |   80   DSI_D3N  PANTHER_TOP_CTE_DIE_BUMP_0_383  BGA10X10_BGA_B2
   A2   |   81   DSI_D3P  PANTHER_TOP_CTE_DIE_BUMP_0_425  BGA10X10_BGA_A2
   C4   |   82   DSI_REXT  PANTHER_TOP_CTE_DIE_BUMP_0_486  BGA10X10_BGA_C4
   W4   |   83   JTCK_SWCLK  PANTHER_TOP_CTE_DIE_BUMP_0_174  BGA10X10_BGA_W4
   W3   |   84   JTDI  PANTHER_TOP_CTE_DIE_BUMP_0_173  BGA10X10_BGA_W3
   V1   |   85   JTDO_TRACESWO  PANTHER_TOP_CTE_DIE_BUMP_0_197  BGA10X10_BGA_V1
   W2   |   86   JTMS_SWDIO  PANTHER_TOP_CTE_DIE_BUMP_0_198  BGA10X10_BGA_W2
   F1   |   87   LVDS1_D0N  PANTHER_TOP_CTE_DIE_BUMP_0_652  BGA10X10_BGA_F1
   F2   |   88   LVDS1_D0P  PANTHER_TOP_CTE_DIE_BUMP_0_653  BGA10X10_BGA_F2
   F3   |   89   LVDS1_D1N  PANTHER_TOP_CTE_DIE_BUMP_0_644  BGA10X10_BGA_F3
   F4   |   90   LVDS1_D1P  PANTHER_TOP_CTE_DIE_BUMP_0_645  BGA10X10_BGA_F4
   G3   |   91   LVDS1_D2N  PANTHER_TOP_CTE_DIE_BUMP_0_636  BGA10X10_BGA_G3
   G4   |   92   LVDS1_D2P  PANTHER_TOP_CTE_DIE_BUMP_0_637  BGA10X10_BGA_G4
   J2   |   93   LVDS1_D3N  PANTHER_TOP_CTE_DIE_BUMP_0_628  BGA10X10_BGA_J2
   J3   |   94   LVDS1_D3P  PANTHER_TOP_CTE_DIE_BUMP_0_629  BGA10X10_BGA_J3
   H3   |   95   LVDS1_D4N  PANTHER_TOP_CTE_DIE_BUMP_0_620  BGA10X10_BGA_H3
   H4   |   96   LVDS1_D4P  PANTHER_TOP_CTE_DIE_BUMP_0_621  BGA10X10_BGA_H4
   V2   |   97   NJTRST  PANTHER_TOP_CTE_DIE_BUMP_0_149  BGA10X10_BGA_V2
   N2   |   98   NRST  PANTHER_TOP_CTE_DIE_BUMP_0_148  BGA10X10_BGA_N2
   T1   |   99   NRSTC1MS  PANTHER_TOP_CTE_DIE_BUMP_0_146  BGA10X10_BGA_T1
   M2   |   100   OSC32_IN  PANTHER_TOP_CTE_DIE_BUMP_0_541  BGA10X10_BGA_M2
   M1   |   101   OSC32_OUT  PANTHER_TOP_CTE_DIE_BUMP_0_540  BGA10X10_BGA_M1
   R1   |   102   OSC_IN  PANTHER_TOP_CTE_DIE_BUMP_0_23  BGA10X10_BGA_R1
   R2   |   103   OSC_OUT  PANTHER_TOP_CTE_DIE_BUMP_0_48  BGA10X10_BGA_R2
   P15   |   104   PA0  PANTHER_TOP_CTE_DIE_BUMP_0_45  BGA10X10_BGA_P15
   N15   |   105   PA1  PANTHER_TOP_CTE_DIE_BUMP_0_9  BGA10X10_BGA_N15
   N12   |   106   PA2  PANTHER_TOP_CTE_DIE_BUMP_0_133  BGA10X10_BGA_N12
   R12   |   107   PA3  PANTHER_TOP_CTE_DIE_BUMP_0_59  BGA10X10_BGA_R12
   P12   |   108   PA4  PANTHER_TOP_CTE_DIE_BUMP_0_84  BGA10X10_BGA_P12
   J12   |   109   PA5  PANTHER_TOP_CTE_DIE_BUMP_0_10  BGA10X10_BGA_J12
   M14   |   110   PA6  PANTHER_TOP_CTE_DIE_BUMP_0_60  BGA10X10_BGA_M14
   K15   |   111   PA7  PANTHER_TOP_CTE_DIE_BUMP_0_110  BGA10X10_BGA_K15
   K9   |   112   PA8  PANTHER_TOP_CTE_DIE_BUMP_0_35  BGA10X10_BGA_K9
   K12   |   113   PA9  PANTHER_TOP_CTE_DIE_BUMP_0_135  BGA10X10_BGA_K12
   M15   |   114   PA10  PANTHER_TOP_CTE_DIE_BUMP_0_11  BGA10X10_BGA_M15
   R9   |   115   PA11  PANTHER_TOP_CTE_DIE_BUMP_0_36  BGA10X10_BGA_R9
   R8   |   116   PA12  PANTHER_TOP_CTE_DIE_BUMP_0_86  BGA10X10_BGA_R8
   W9   |   117   PA13  PANTHER_TOP_CTE_DIE_BUMP_0_136  BGA10X10_BGA_W9
   T8   |   118   PA14  PANTHER_TOP_CTE_DIE_BUMP_0_12  BGA10X10_BGA_T8
   T10   |   119   PA15  PANTHER_TOP_CTE_DIE_BUMP_0_62  BGA10X10_BGA_T10
   B8   |   120   PB0  PANTHER_TOP_CTE_DIE_BUMP_0_464  BGA10X10_BGA_B8
   D9   |   121   PB1  PANTHER_TOP_CTE_DIE_BUMP_0_485  BGA10X10_BGA_D9
   E9   |   122   PB2  PANTHER_TOP_CTE_DIE_BUMP_0_401  BGA10X10_BGA_E9
   A9   |   123   PB3  PANTHER_TOP_CTE_DIE_BUMP_0_443  BGA10X10_BGA_A9
   C9   |   124   PB4  PANTHER_TOP_CTE_DIE_BUMP_0_463  BGA10X10_BGA_C9
   B9   |   125   PB5  PANTHER_TOP_CTE_DIE_BUMP_0_421  BGA10X10_BGA_B9
   C8   |   126   PB6  PANTHER_TOP_CTE_DIE_BUMP_0_442  BGA10X10_BGA_C8
   D7   |   127   PB7  PANTHER_TOP_CTE_DIE_BUMP_0_484  BGA10X10_BGA_D7
   A7   |   128   PB8  PANTHER_TOP_CTE_DIE_BUMP_0_420  BGA10X10_BGA_A7
   A8   |   129   PB9  PANTHER_TOP_CTE_DIE_BUMP_0_378  BGA10X10_BGA_A8
   E12   |   130   PB10  PANTHER_TOP_CTE_DIE_BUMP_0_462  BGA10X10_BGA_E12
   B7   |   131   PB11  PANTHER_TOP_CTE_DIE_BUMP_0_483  BGA10X10_BGA_B7
   E14   |   132   PB12  PANTHER_TOP_CTE_DIE_BUMP_0_391  BGA10X10_BGA_E14
   G15   |   133   PB13  PANTHER_TOP_CTE_DIE_BUMP_0_453  BGA10X10_BGA_G15
   H15   |   134   PB14  PANTHER_TOP_CTE_DIE_BUMP_0_390  BGA10X10_BGA_H15
   J15   |   135   PB15  PANTHER_TOP_CTE_DIE_BUMP_0_20  BGA10X10_BGA_J15
   V9   |   136   PC0  PANTHER_TOP_CTE_DIE_BUMP_0_137  BGA10X10_BGA_V9
   V10   |   137   PC1  PANTHER_TOP_CTE_DIE_BUMP_0_13  BGA10X10_BGA_V10
   T9   |   138   PC2  PANTHER_TOP_CTE_DIE_BUMP_0_63  BGA10X10_BGA_T9
   U4   |   139   PC3  PANTHER_TOP_CTE_DIE_BUMP_0_139  BGA10X10_BGA_U4
   V3   |   140   PC4  PANTHER_TOP_CTE_DIE_BUMP_0_115  BGA10X10_BGA_V3
   T7   |   141   PC5  PANTHER_TOP_CTE_DIE_BUMP_0_65  BGA10X10_BGA_T7
   R7   |   142   PC6  PANTHER_TOP_CTE_DIE_BUMP_0_140  BGA10X10_BGA_R7
   W5   |   143   PC7  PANTHER_TOP_CTE_DIE_BUMP_0_40  BGA10X10_BGA_W5
   U6   |   144   PC8  PANTHER_TOP_CTE_DIE_BUMP_0_16  BGA10X10_BGA_U6
   V6   |   145   PC9  PANTHER_TOP_CTE_DIE_BUMP_0_66  BGA10X10_BGA_V6
   W6   |   146   PC10  PANTHER_TOP_CTE_DIE_BUMP_0_116  BGA10X10_BGA_W6
   V5   |   147   PC11  PANTHER_TOP_CTE_DIE_BUMP_0_117  BGA10X10_BGA_V5
   V4   |   148   PC12  PANTHER_TOP_CTE_DIE_BUMP_0_119  BGA10X10_BGA_V4
   P4   |   149   PC13  PANTHER_TOP_CTE_DIE_BUMP_0_199  BGA10X10_BGA_P4
   V13   |   150   PCIE_CLKINN  PANTHER_TOP_CTE_DIE_BUMP_0_76  BGA10X10_BGA_V13
   U13   |   151   PCIE_CLKINP  PANTHER_TOP_CTE_DIE_BUMP_0_26  BGA10X10_BGA_U13
   V14   |   152   PCIE_CLKOUTN  PANTHER_TOP_CTE_DIE_BUMP_0_27  BGA10X10_BGA_V14
   U14   |   153   PCIE_CLKOUTP  PANTHER_TOP_CTE_DIE_BUMP_TEST_945  BGA10X10_BGA_U14
   C11   |   154   PD0  PANTHER_TOP_CTE_DIE_BUMP_0_482  BGA10X10_BGA_C11
   F9   |   155   PD1  PANTHER_TOP_CTE_DIE_BUMP_0_440  BGA10X10_BGA_F9
   A10   |   156   PD2  PANTHER_TOP_CTE_DIE_BUMP_0_398  BGA10X10_BGA_A10
   D8   |   157   PD3  PANTHER_TOP_CTE_DIE_BUMP_0_460  BGA10X10_BGA_D8
   C12   |   158   PD4  PANTHER_TOP_CTE_DIE_BUMP_0_418  BGA10X10_BGA_C12
   B12   |   159   PD5  PANTHER_TOP_CTE_DIE_BUMP_0_376  BGA10X10_BGA_B12
   A12   |   160   PD6  PANTHER_TOP_CTE_DIE_BUMP_0_481  BGA10X10_BGA_A12
   D12   |   161   PD7  PANTHER_TOP_CTE_DIE_BUMP_0_459  BGA10X10_BGA_D12
   E11   |   162   PD8  PANTHER_TOP_CTE_DIE_BUMP_0_375  BGA10X10_BGA_E11
   C10   |   163   PD9  PANTHER_TOP_CTE_DIE_BUMP_0_417  BGA10X10_BGA_C10
   D11   |   164   PD10  PANTHER_TOP_CTE_DIE_BUMP_0_480  BGA10X10_BGA_D11
   B10   |   165   PD11  PANTHER_TOP_CTE_DIE_BUMP_0_438  BGA10X10_BGA_B10
   H14   |   166   PD12  PANTHER_TOP_CTE_DIE_BUMP_0_389  BGA10X10_BGA_H14
   G9   |   167   PD13  PANTHER_TOP_CTE_DIE_BUMP_0_431  BGA10X10_BGA_G9
   A13   |   168   PD14  PANTHER_TOP_CTE_DIE_BUMP_0_351  BGA10X10_BGA_A13
   A11   |   169   PD15  PANTHER_TOP_CTE_DIE_BUMP_0_367  BGA10X10_BGA_A11
   N1   |   170   PDR_ON  PANTHER_TOP_CTE_DIE_BUMP_0_585  BGA10X10_BGA_N1
   B13   |   171   PE0  PANTHER_TOP_CTE_DIE_BUMP_0_458  BGA10X10_BGA_B13
   C13   |   172   PE1  PANTHER_TOP_CTE_DIE_BUMP_0_479  BGA10X10_BGA_C13
   A14   |   173   PE2  PANTHER_TOP_CTE_DIE_BUMP_0_395  BGA10X10_BGA_A14
   A15   |   174   PE3  PANTHER_TOP_CTE_DIE_BUMP_0_437  BGA10X10_BGA_A15
   B14   |   175   PE4  PANTHER_TOP_CTE_DIE_BUMP_0_457  BGA10X10_BGA_B14
   C14   |   176   PE5  PANTHER_TOP_CTE_DIE_BUMP_0_415  BGA10X10_BGA_C14
   F14   |   177   PE6  PANTHER_TOP_CTE_DIE_BUMP_0_478  BGA10X10_BGA_F14
   C15   |   178   PE7  PANTHER_TOP_CTE_DIE_BUMP_0_414  BGA10X10_BGA_C15
   B15   |   179   PE8  PANTHER_TOP_CTE_DIE_BUMP_0_456  BGA10X10_BGA_B15
   F15   |   180   PE9  PANTHER_TOP_CTE_DIE_BUMP_0_393  BGA10X10_BGA_F15
   D15   |   181   PE10  PANTHER_TOP_CTE_DIE_BUMP_0_435  BGA10X10_BGA_D15
   B16   |   182   PE11  PANTHER_TOP_CTE_DIE_BUMP_0_477  BGA10X10_BGA_B16
   C16   |   183   PE12  PANTHER_TOP_CTE_DIE_BUMP_0_455  BGA10X10_BGA_C16
   A16   |   184   PE13  PANTHER_TOP_CTE_DIE_BUMP_0_392  BGA10X10_BGA_A16
   G14   |   185   PE14  PANTHER_TOP_CTE_DIE_BUMP_0_434  BGA10X10_BGA_G14
   D14   |   186   PE15  PANTHER_TOP_CTE_DIE_BUMP_0_476  BGA10X10_BGA_D14
   N9   |   187   PF0  PANTHER_TOP_CTE_DIE_BUMP_0_88  BGA10X10_BGA_N9
   U8   |   188   PF1  PANTHER_TOP_CTE_DIE_BUMP_0_138  BGA10X10_BGA_U8
   P9   |   189   PF2  PANTHER_TOP_CTE_DIE_BUMP_0_64  BGA10X10_BGA_P9
   W10   |   190   PF3  PANTHER_TOP_CTE_DIE_BUMP_0_14  BGA10X10_BGA_W10
   W7   |   191   PF4  PANTHER_TOP_CTE_DIE_BUMP_0_114  BGA10X10_BGA_W7
   P7   |   192   PF5  PANTHER_TOP_CTE_DIE_BUMP_0_89  BGA10X10_BGA_P7
   U5   |   193   PF6  PANTHER_TOP_CTE_DIE_BUMP_0_39  BGA10X10_BGA_U5
   V7   |   194   PF7  PANTHER_TOP_CTE_DIE_BUMP_0_15  BGA10X10_BGA_V7
   U7   |   195   PF8  PANTHER_TOP_CTE_DIE_BUMP_0_90  BGA10X10_BGA_U7
   T6   |   196   PF9  PANTHER_TOP_CTE_DIE_BUMP_0_118  BGA10X10_BGA_T6
   L9   |   197   PF10  PANTHER_TOP_CTE_DIE_BUMP_0_19  BGA10X10_BGA_L9
   T4   |   198   PF11  PANTHER_TOP_CTE_DIE_BUMP_0_144  BGA10X10_BGA_T4
   L7   |   199   PF12  PANTHER_TOP_CTE_DIE_BUMP_0_576  BGA10X10_BGA_L7
   H2   |   200   PF13  PANTHER_TOP_CTE_DIE_BUMP_0_581  BGA10X10_BGA_H2
   G7   |   201   PF14  PANTHER_TOP_CTE_DIE_BUMP_0_582  BGA10X10_BGA_G7
   G5   |   202   PF15  PANTHER_TOP_CTE_DIE_BUMP_0_586  BGA10X10_BGA_G5
   T5   |   203   PG0  PANTHER_TOP_CTE_DIE_BUMP_0_69  BGA10X10_BGA_T5
   R4   |   204   PG1  PANTHER_TOP_CTE_DIE_BUMP_0_94  BGA10X10_BGA_R4
   M7   |   205   PG2  PANTHER_TOP_CTE_DIE_BUMP_0_44  BGA10X10_BGA_M7
   H12   |   206   PG3  PANTHER_TOP_CTE_DIE_BUMP_0_120  BGA10X10_BGA_H12
   N7   |   207   PG4  PANTHER_TOP_CTE_DIE_BUMP_0_70  BGA10X10_BGA_N7
   K1   |   208   PG5  PANTHER_TOP_CTE_DIE_BUMP_0_588  BGA10X10_BGA_K1
   K2   |   209   PG6  PANTHER_TOP_CTE_DIE_BUMP_0_589  BGA10X10_BGA_K2
   E7   |   210   PG7  PANTHER_TOP_CTE_DIE_BUMP_0_590  BGA10X10_BGA_E7
   E5   |   211   PG8  PANTHER_TOP_CTE_DIE_BUMP_0_592  BGA10X10_BGA_E5
   G2   |   212   PG9  PANTHER_TOP_CTE_DIE_BUMP_0_596  BGA10X10_BGA_G2
   F5   |   213   PG10  PANTHER_TOP_CTE_DIE_BUMP_0_597  BGA10X10_BGA_F5
   F7   |   214   PG11  PANTHER_TOP_CTE_DIE_BUMP_0_598  BGA10X10_BGA_F7
   H7   |   215   PG12  PANTHER_TOP_CTE_DIE_BUMP_0_600  BGA10X10_BGA_H7
   J7   |   216   PG13  PANTHER_TOP_CTE_DIE_BUMP_0_601  BGA10X10_BGA_J7
   H5   |   217   PG14  PANTHER_TOP_CTE_DIE_BUMP_0_602  BGA10X10_BGA_H5
   E4   |   218   PG15  PANTHER_TOP_CTE_DIE_BUMP_0_606  BGA10X10_BGA_E4
   L14   |   219   PH2  PANTHER_TOP_CTE_DIE_BUMP_0_83  BGA10X10_BGA_L14
   K14   |   220   PH3  PANTHER_TOP_CTE_DIE_BUMP_0_109  BGA10X10_BGA_K14
   G12   |   221   PH4  PANTHER_TOP_CTE_DIE_BUMP_0_34  BGA10X10_BGA_G12
   M9   |   222   PH5  PANTHER_TOP_CTE_DIE_BUMP_0_134  BGA10X10_BGA_M9
   L15   |   223   PH6  PANTHER_TOP_CTE_DIE_BUMP_0_85  BGA10X10_BGA_L15
   L12   |   224   PH7  PANTHER_TOP_CTE_DIE_BUMP_0_61  BGA10X10_BGA_L12
   M12   |   225   PH8  PANTHER_TOP_CTE_DIE_BUMP_0_111  BGA10X10_BGA_M12
   W8   |   226   PH9  PANTHER_TOP_CTE_DIE_BUMP_0_112  BGA10X10_BGA_W8
   U10   |   227   PH10  PANTHER_TOP_CTE_DIE_BUMP_0_87  BGA10X10_BGA_U10
   T11   |   228   PH11  PANTHER_TOP_CTE_DIE_BUMP_0_37  BGA10X10_BGA_T11
   V8   |   229   PH12  PANTHER_TOP_CTE_DIE_BUMP_0_113  BGA10X10_BGA_V8
   U9   |   230   PH13  PANTHER_TOP_CTE_DIE_BUMP_0_38  BGA10X10_BGA_U9
   H1   |   231   PI0  PANTHER_TOP_CTE_DIE_BUMP_0_605  BGA10X10_BGA_H1
   J9   |   232   PI1  PANTHER_TOP_CTE_DIE_BUMP_0_604  BGA10X10_BGA_J9
   J5   |   233   PI2  PANTHER_TOP_CTE_DIE_BUMP_0_608  BGA10X10_BGA_J5
   H9   |   234   PI3  PANTHER_TOP_CTE_DIE_BUMP_0_609  BGA10X10_BGA_H9
   G1   |   235   PI4  PANTHER_TOP_CTE_DIE_BUMP_0_610  BGA10X10_BGA_G1
   K7   |   236   PI5  PANTHER_TOP_CTE_DIE_BUMP_0_614  BGA10X10_BGA_K7
   D4   |   237   PI6  PANTHER_TOP_CTE_DIE_BUMP_0_613  BGA10X10_BGA_D4
   D5   |   238   PI7  PANTHER_TOP_CTE_DIE_BUMP_0_612  BGA10X10_BGA_D5
   N4   |   239   PI8  PANTHER_TOP_CTE_DIE_BUMP_0_536  BGA10X10_BGA_N4
   K6   |   240   PI9  PANTHER_TOP_CTE_DIE_BUMP_0_618  BGA10X10_BGA_K6
   B11   |   241   PI10  PANTHER_TOP_CTE_DIE_BUMP_0_411  BGA10X10_BGA_B11
   F12   |   242   PI11  PANTHER_TOP_CTE_DIE_BUMP_0_359  BGA10X10_BGA_F12
   P2   |   243   PWR_CPUON  PANTHER_TOP_CTE_DIE_BUMP_0_74  BGA10X10_BGA_P2
   P1   |   244   PWR_LP  PANTHER_TOP_CTE_DIE_BUMP_0_99  BGA10X10_BGA_P1
   U3   |   245   PWR_ON  PANTHER_TOP_CTE_DIE_BUMP_0_98  BGA10X10_BGA_U3
   L5   |   246   PZ0  PANTHER_TOP_CTE_DIE_BUMP_0_556  BGA10X10_BGA_L5
   M4   |   247   PZ1  PANTHER_TOP_CTE_DIE_BUMP_0_554  BGA10X10_BGA_M4
   M3   |   248   PZ2  PANTHER_TOP_CTE_DIE_BUMP_0_557  BGA10X10_BGA_M3
   M5   |   249   PZ3  PANTHER_TOP_CTE_DIE_BUMP_0_558  BGA10X10_BGA_M5
   L4   |   250   PZ4  PANTHER_TOP_CTE_DIE_BUMP_0_562  BGA10X10_BGA_L4
   N3   |   251   PZ5  PANTHER_TOP_CTE_DIE_BUMP_0_561  BGA10X10_BGA_N3
   K3   |   252   PZ6  PANTHER_TOP_CTE_DIE_BUMP_0_560  BGA10X10_BGA_K3
   L1   |   253   PZ7  PANTHER_TOP_CTE_DIE_BUMP_0_564  BGA10X10_BGA_L1
   L3   |   254   PZ8  PANTHER_TOP_CTE_DIE_BUMP_0_565  BGA10X10_BGA_L3
   L2   |   255   PZ9  PANTHER_TOP_CTE_DIE_BUMP_0_566  BGA10X10_BGA_L2
   W13   |   256   UCPD1_CC1  PANTHER_TOP_CTE_DIE_BUMP_0_8  BGA10X10_BGA_W13
   W14   |   257   UCPD1_CC2  PANTHER_TOP_CTE_DIE_BUMP_0_32  BGA10X10_BGA_W14
   V12   |   258   USB3DR_DM  PANTHER_TOP_CTE_DIE_BUMP_0_54  BGA10X10_BGA_V12
   W12   |   259   USB3DR_DP  PANTHER_TOP_CTE_DIE_BUMP_0_28  BGA10X10_BGA_W12
   R15   |   260   USB3DR_TXRTUNE  PANTHER_TOP_CTE_DIE_BUMP_0_29  BGA10X10_BGA_R15
   T12   |   261   USB3DR_VBUS  PANTHER_TOP_CTE_DIE_BUMP_0_53  BGA10X10_BGA_T12
   V11   |   262   USBH_HS_DM  PANTHER_TOP_CTE_DIE_BUMP_0_56  BGA10X10_BGA_V11
   W11   |   263   USBH_HS_DP  PANTHER_TOP_CTE_DIE_BUMP_0_30  BGA10X10_BGA_W11
   T15   |   264   USBH_HS_TXRTUNE  PANTHER_TOP_CTE_DIE_BUMP_0_31  BGA10X10_BGA_T15
   M8   |   265   V08CAP  PANTHER_TOP_CTE_DIE_BUMP_0_551  BGA10X10_BGA_M8
   R6   |   266   VBAT  PANTHER_TOP_CTE_DIE_BUMP_0_549  BGA10X10_BGA_R6
   U11   |   267   VDD33UCPD  PANTHER_TOP_CTE_DIE_BUMP_0_7  BGA10X10_BGA_U11
   R14   |   268   VDD33USB  PANTHER_TOP_CTE_DIE_BUMP_0_104  BGA10X10_BGA_R14
   K8   |   269   VDD  PANTHER_TOP_CTE_DIE_BUMP_0_575  BGA10X10_BGA_K8
   N6   |   270   VDDA18ADC  PANTHER_TOP_CTE_DIE_BUMP_0_41  BGA10X10_BGA_N6
   N5   |   271   VDDA18AON  PANTHER_TOP_CTE_DIE_BUMP_0_366  BGA10X10_BGA_N5
   R13   |   272   VDDA18COMBOPHY  PANTHER_TOP_CTE_DIE_BUMP_0_102  BGA10X10_BGA_R13
   D3   |   273   VDDA18CSI  PANTHER_TOP_CTE_DIE_BUMP_0_447  BGA10X10_BGA_D3
   D16   |   274   VDDA18DDR  PANTHER_TOP_CTE_DIE_BUMP_0_278  BGA10X10_BGA_D16
   C5   |   275   VDDA18DSI  PANTHER_TOP_CTE_DIE_BUMP_0_444  BGA10X10_BGA_C5
   J4   |   276   VDDA18LVDS  PANTHER_TOP_CTE_DIE_BUMP_0_640  BGA10X10_BGA_J4
   E15   |   277   VDDA18PLL1  PANTHER_TOP_CTE_DIE_CENTRAL_BUMP_839  BGA10X10_BGA_E15
   G6   |   278   VDDA18PLL2  PANTHER_TOP_CTE_DIE_BUMP_CEN_941  BGA10X10_BGA_G6
   H6   |   279   VDDA18PLL3  PANTHER_TOP_CTE_DIE_BUMP_CEN_942  BGA10X10_BGA_H6
   T13   |   280   VDDA18USB  PANTHER_TOP_CTE_DIE_BUMP_0_80  BGA10X10_BGA_T13
   T14   |   281   VDDCOMBOPHY  PANTHER_TOP_CTE_DIE_BUMP_0_126  BGA10X10_BGA_T14
   W16   |   282   VDDCOMBOPHYTX  PANTHER_TOP_CTE_DIE_BUMP_0_101  BGA10X10_BGA_W16
   J10   |   283   VDDCORE  PANTHER_TOP_CTE_DIE_CENTRAL_BUMP_9231  BGA10X10_BGA_J10
   J13   |   284   VDDCPU  PANTHER_TOP_CTE_DIE_CENTRAL_BUMP_819  BGA10X10_BGA_J13
   B1   |   285   VDDCSI  PANTHER_TOP_CTE_DIE_BUMP_0_468  BGA10X10_BGA_B1
   C6   |   286   VDDDSI  PANTHER_TOP_CTE_DIE_BUMP_0_465  BGA10X10_BGA_C6
   M11   |   287   VDDGPU  PANTHER_TOP_CTE_DIE_CENTRAL_BUMP_9372  BGA10X10_BGA_M11
   D10   |   288   VDDIO1  PANTHER_TOP_CTE_DIE_BUMP_0_373  BGA10X10_BGA_D10
   F8   |   289   VDDIO2  PANTHER_TOP_CTE_DIE_BUMP_0_371  BGA10X10_BGA_F8
   E10   |   290   VDDIO3  PANTHER_TOP_CTE_DIE_BUMP_0_397  BGA10X10_BGA_E10
   E6   |   291   VDDIO4  PANTHER_TOP_CTE_DIE_BUMP_0_399  BGA10X10_BGA_E6
   J1   |   292   VDDLVDS  PANTHER_TOP_CTE_DIE_BUMP_0_670  BGA10X10_BGA_J1
   U12   |   293   VDDPCIECLK  PANTHER_TOP_CTE_DIE_BUMP_0_127  BGA10X10_BGA_U12
   T16   |   294   VDDQDDR  PANTHER_TOP_CTE_DIE_BUMP_0_282  BGA10X10_BGA_T16
   U1   |   295   VREFN  PANTHER_TOP_CTE_DIE_BUMP_0_68  BGA10X10_BGA_U1
   U2   |   296   VREFP  PANTHER_TOP_CTE_DIE_BUMP_0_18  BGA10X10_BGA_U2
   C7   |   297   VSS  PANTHER_TOP_CTE_DIE_CENTRAL_BUMP_9252  BGA10X10_BGA_C7
   P6   |   298   VSSA  PANTHER_TOP_CTE_DIE_BUMP_0_92  BGA10X10_BGA_P6
   M6   |   299   VSSAON  PANTHER_TOP_CTE_DIE_BUMP_0_552  BGA10X10_BGA_M6
[Model Data]
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[End Model Data]
[End Package Model]
|[End]
|End [Component]
| Models and submodels in the file (84): synopsys_usb3_tx (Output), synopsys_usb3_rx (Input), USB2_HSRX (Input), USB2_HSTX_00_0_01_0011_11 (Output), USB2_HSTX_00_0_10_0101_11 (Output), USB2_HSTX_00_0_11_0111_11 (Output), USB2_HSTX_00_1_01_0011_11 (Output), USB2_HSTX_00_1_10_0101_11 (Output), USB2_HSTX_00_1_11_0111_11 (Output), USB2_HSTX_01_0_01_0011_11 (Output), USB2_HSTX_01_0_10_0101_11 (Output), USB2_HSTX_01_0_11_0111_11 (Output), USB2_HSTX_01_1_01_0011_11 (Output), USB2_HSTX_01_1_10_0101_11 (Output), USB2_HSTX_01_1_11_0111_11 (Output), USB2_HSTX_10_0_01_0011_11 (Output), USB2_HSTX_10_0_10_0101_11 (Output), USB2_HSTX_10_0_11_0111_11 (Output), USB2_HSTX_10_1_01_0011_11 (Output), USB2_HSTX_10_1_10_0101_11 (Output), USB2_HSTX_10_1_11_0111_11 (Output), DPHY_TX_2P5G (Output), DPHY_TX_1P5G (Output), DPHY_RX_1P5G_L1 (Input), DPHY_RX_2P5G_L1 (Input), io8_tt_fs_3v3 (I/O), io8_tt_hs_3v3 (I/O), io8_tt_hslv_fs_1v8 (I/O), io8_tt_hslv_hs_1v8 (I/O), io8_tt_hslv_ls_1v8 (I/O), io8_tt_hslv_ms_1v8 (I/O), io8_tt_i3c_3v3 (I/O_open_drain), io8_tt_ls_3v3 (I/O), io8_tt_ms_3v3 (I/O), isudq_tt_1v8 (Input), isudq_tt_3v3 (Input), mal4drv20_d3_20 (I/O), mal4drv20_d3_24 (I/O), mal4drv20_d3_30 (I/O), mal4drv20_d3_40 (I/O), mal4drv20_d3_60 (I/O), mal4drv20_d4_20 (I/O), mal4drv20_d4_24 (I/O), mal4drv20_d4_30 (I/O), mal4drv20_d4_40 (I/O), mal4drv20_d4_60 (I/O), mal4drv20_dl4_20 (I/O), mal4drv20_dl4_24 (I/O), mal4drv20_dl4_30 (I/O), mal4drv20_dl4_40 (I/O), mal4drv20_dl4_60 (I/O), mal4drv27_d3_28 (I/O), mal4drv27_d3_34 (I/O), mal4drv27_d3_40 (I/O), mal4drv27_d3_53 (I/O), mal4drv27_d3_odt120 (Input), mal4drv27_d3_odt60 (Input), mal4drv27_dl4_28 (I/O), mal4drv27_dl4_34 (I/O), mal4drv27_dl4_40 (I/O), mal4drv27_dl4_53 (I/O), mal4drv27_dl4_odt48 (Input), mal4drv27_dl4_odt60 (Input), mal4drv27_d4_28 (I/O), mal4drv27_d4_34 (I/O), mal4drv27_d4_40 (I/O), mal4drv27_d4_53 (I/O), mal4drv27_d4_odt120 (Input), mal4drv27_d4_odt240 (Input), mal4drv27_d4_odt48 (Input), mal4drv27_d4_odt60 (Input), mal4drv27_d4_odt80 (Input), mal4drv20_d3l_120 (I/O), mal4drv20_d3l_40 (I/O), mal4drv20_d3l_60 (I/O), mal4drv27_d3l_120 (I/O), mal4drv27_d3l_240 (I/O), mal4drv27_d3l_40 (I/O), mal4drv27_d3l_48 (I/O), mal4drv27_d3l_60 (I/O)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
